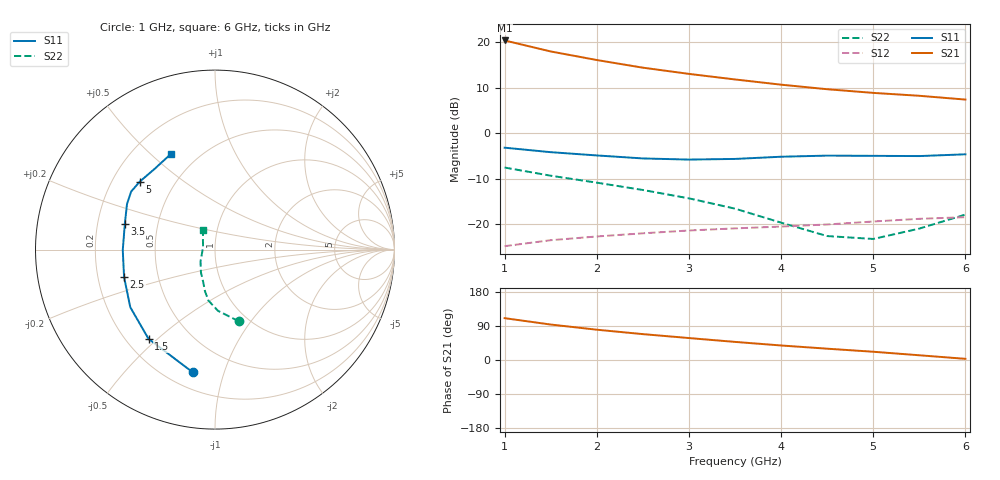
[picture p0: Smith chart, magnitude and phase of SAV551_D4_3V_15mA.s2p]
! Created Mon Oct 27 14:25:00 2008
# hz S ma R 50
! 2 Port Network Data from SP1.SP block
! freq  magS11  angS11  magS21  angS21  magS12  angS12  magS22  angS22
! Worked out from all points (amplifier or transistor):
!   11 points, 1 GHz to 6 GHz, reference 50 ohm
!   highest |S21| = 20.4 dB at 1 GHz (marker M1)
!   |S21| within 3 dB of that: start of sweep to 1.654 GHz
!   unconditionally stable (mu >= 1): 2.93 GHz to end of sweep
!   at 1.5 GHz: K = 0.58, MSG = 20.8 dB, |S12| = -23.5 dB
!   at 3.5 GHz: K = 1.11, MAG = 14.3 dB, |S12| = -20.9 dB
!   at 6 GHz: K = 1.33, MAG = 9.5 dB, |S12| = -18.5 dB
!   S11 on the Smith chart (normalised r, x): 1 GHz: 0.30, -0.79; 1.5 GHz: 0.29, -0.47; 2.5 GHz: 0.31, -0.13; 3.5 GHz: 0.32, +0.13; 5 GHz: 0.32, +0.35; 6 GHz: 0.36, +0.58
1e9  0.6946 -100.3  10.5 110.4  0.05733 38.0  0.4201 -71.7
1.5e9  0.62 -126.7  7.949 93.6  0.06669 30.1  0.3415 -87.2
2e9  0.5708 -145.8  6.398 79.9  0.07329 24.1  0.2864 -97.4
2.5e9  0.529 -163.3  5.271 68.3  0.07941 20.3  0.2379 -103.6
3e9  0.5139 -179.7  4.503 57.9  0.08527 17.2  0.1926 -110.0
3.5e9  0.5225 164.1  3.911 47.8  0.08997 13.3  0.1483 -121.9
4e9  0.5523 152.5  3.427 38.3  0.0942 10.5  0.104 -140.8
4.5e9  0.5682 145.3  3.054 29.8  0.09931 8.4  0.07407 -166.3
5e9  0.5649 137.9  2.783 21.8  0.1071 5.5  0.0688 165.2
5.5e9  0.5616 126.8  2.586 12.5  0.1146 1.2  0.0895 138.8
6e9  0.5873 114.6  2.35 3.1  0.1195 -3.3  0.1276 121.3
